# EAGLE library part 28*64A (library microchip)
CMOS EEPROM 64 K (8 K x 8), low voltage
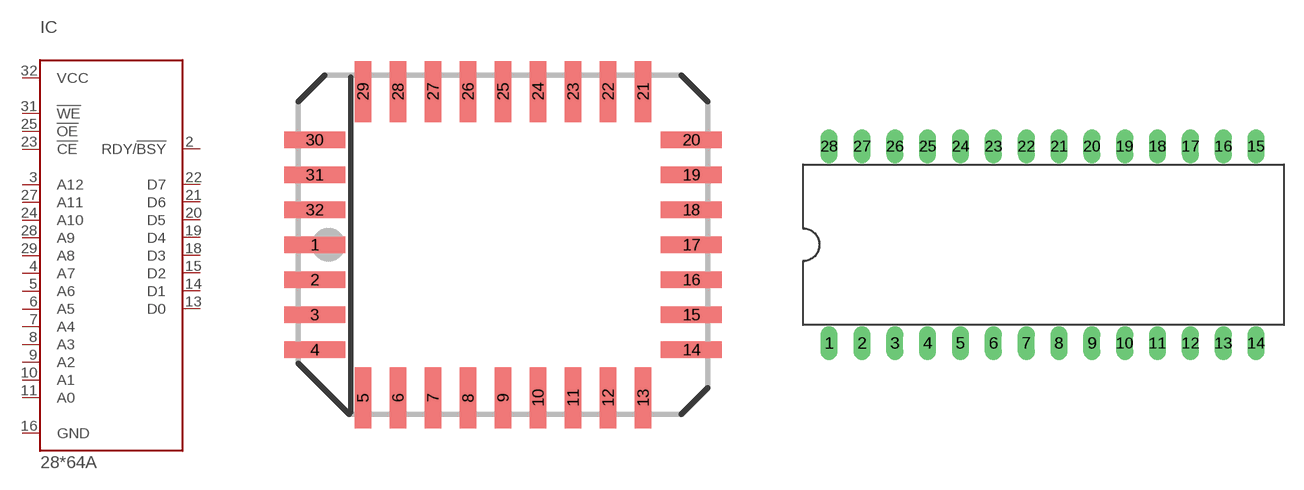
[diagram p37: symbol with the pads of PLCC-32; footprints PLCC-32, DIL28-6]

Designator prefix IC

## 28C64AL (MPN: CAT28C64BGI-12T; OC_FARNELL: 1718494; OC_NEWARK: 08R5439), 28VL64AL (OC_FARNELL: unknown; OC_NEWARK: unknown)  [PLCC-32]
2  RDY/!BSY  out
3  A12  in
4  A7  in
5  A6  in
6  A5  in
7  A4  in
8  A3  in
9  A2  in
10  A1  in
11  A0  in
13  D0  hiz
14  D1  hiz
15  D2  hiz
16  GND  pwr
18  D3  hiz
19  D4  hiz
20  D5  hiz
21  D6  hiz
22  D7  hiz
23  !CE  in
24  A10  in
25  !OE  in
27  A11  in
28  A9  in
29  A8  in
31  !WE  in
32  VCC  pwr

## 28C64AP (MPN: AT28C64B-15PU; OC_FARNELL: 1631144; OC_NEWARK: 96K6557), 28LV64AP (MPN: CAT28LV64LI-25; OC_FARNELL: unknown; OC_NEWARK: 06R0912)  [DIL28-6]
1  RDY/!BSY  out
2  A12  in
3  A7  in
4  A6  in
5  A5  in
6  A4  in
7  A3  in
8  A2  in
9  A1  in
10  A0  in
11  D0  hiz
12  D1  hiz
13  D2  hiz
14  GND  pwr
15  D3  hiz
16  D4  hiz
17  D5  hiz
18  D6  hiz
19  D7  hiz
20  !CE  in
21  A10  in
22  !OE  in
23  A11  in
24  A9  in
25  A8  in
27  !WE  in
28  VCC  pwr

## 28C64ASO (MPN: CAT28C64BWI-12; OC_FARNELL: 1718312; OC_NEWARK: 06R0739), 28LV64ASO (MPN: CAT28LV64W-25; OC_FARNELL: 1718338; OC_NEWARK: 06R0915)  [SO28W]
Pads as for DIL28-6

## 28C64AVS (OC_FARNELL: unknown; OC_NEWARK: unknown), 28LV64AVS (OC_FARNELL: unknown; OC_NEWARK: unknown)  [VSOP28-8X13]
Pads as for DIL28-6

## 28C64ATS (OC_FARNELL: unknown; OC_NEWARK: unknown), 28LV64ATS (MPN: CAT28LV64H13-20; OC_FARNELL: 1718417; OC_NEWARK: 06R0901)  [TSOP28]
1  !OE  in
2  A11  in
3  A9  in
4  A8  in
6  !WE  in
7  VCC  pwr
8  RDY/!BSY  out
9  A12  in
10  A7  in
11  A6  in
12  A5  in
13  A4  in
14  A3  in
15  A2  in
16  A1  in
17  A0  in
18  D0  hiz
19  D1  hiz
20  D2  hiz
21  GND  pwr
22  D3  hiz
23  D4  hiz
24  D5  hiz
25  D6  hiz
26  D7  hiz
27  !CE  in
28  A10  in

## Footprint PLCC-32 (pad centres in mm)
PLASTIC LEADED CHIP CARRIER rectangle, package type L
smd 2.2 x 0.6: 1 -6.83,0; 2 -6.83,-1.27; 3 -6.83,-2.54; 4 -6.83,-3.81; 14 6.83,-3.81; 15 6.83,-2.54; 16 6.83,-1.27; 17 6.83,0; 18 6.83,1.27; 19 6.83,2.54; 20 6.83,3.81; 30 -6.83,3.81; 31 -6.83,2.54; 32 -6.83,1.27
smd 0.6 x 2.2: 5 -5.08,-5.56; 6 -3.81,-5.56; 7 -2.54,-5.56; 8 -1.27,-5.56; 9 0,-5.56; 10 1.27,-5.56; 11 2.54,-5.56; 12 3.81,-5.56; 13 5.08,-5.56; 21 5.08,5.56; 22 3.81,5.56; 23 2.54,5.56; 24 1.27,5.56; 25 0,5.56; 26 -1.27,5.56; 27 -2.54,5.56; 28 -3.81,5.56; 29 -5.08,5.56

## Footprint DIL28-6 (pad centres in mm)
Dual In Line package type P
drill 0.813 long: 1 -16.51,-7.62; 2 -13.97,-7.62; 3 -11.43,-7.62; 4 -8.89,-7.62; 5 -6.35,-7.62; 6 -3.81,-7.62; 7 -1.27,-7.62; 8 1.27,-7.62; 9 3.81,-7.62; 10 6.35,-7.62; 11 8.89,-7.62; 12 11.43,-7.62; 13 13.97,-7.62; 14 16.51,-7.62; 15 16.51,7.62; 16 13.97,7.62; 17 11.43,7.62; 18 8.89,7.62; 19 6.35,7.62; 20 3.81,7.62; 21 1.27,7.62; 22 -1.27,7.62; 23 -3.81,7.62; 24 -6.35,7.62; 25 -8.89,7.62; 26 -11.43,7.62; 27 -13.97,7.62; 28 -16.51,7.62

## Footprint SO28W (pad centres in mm)
28-Lead Plastic Small Outline (SO) Wide, 300 mil Body (SOIC) Source: http://ww1.microchip.com/downloads/en/devicedoc/39632c.pdf
smd 0.65 x 1.7: 1 -7.62,-4.78; 2 -6.35,-4.78; 3 -5.08,-4.78; 4 -3.81,-4.78; 5 -2.54,-4.78; 6 -1.27,-4.78; 7 0,-4.78; 8 1.27,-4.78; 9 2.54,-4.78; 10 3.81,-4.78; 11 5.08,-4.78; 12 6.35,-4.78; 13 7.62,-4.78; 14 8.89,-4.78; 15 8.89,4.78; 16 7.62,4.78; 17 6.35,4.78; 18 5.08,4.78; 19 3.81,4.78; 20 2.54,4.78; 21 1.27,4.78; 22 0,4.78; 23 -1.27,4.78; 24 -2.54,4.78; 25 -3.81,4.78; 26 -5.08,4.78; 27 -6.35,4.78; 28 -7.62,4.78

## Footprint VSOP28-8X13 (pad centres in mm)
Very Small Outline Package 8 x 13.4 mm, package type VS
smd 0.3 x 1.1: 1 0.275,-6.45; 2 0.825,-6.45; 3 1.375,-6.45; 4 1.925,-6.45; 5 2.475,-6.45; 6 3.025,-6.45; 7 3.575,-6.45; 8 3.575,6.45; 9 3.025,6.45; 10 2.475,6.45; 11 1.925,6.45; 12 1.375,6.45; 13 0.825,6.45; 14 0.275,6.45; 15 -0.275,6.45; 16 -0.825,6.45; 17 -1.375,6.45; 18 -1.925,6.45; 19 -2.475,6.45; 20 -3.025,6.45; 21 -3.575,6.45; 22 -3.575,-6.45; 23 -3.025,-6.45; 24 -2.475,-6.45; 25 -1.925,-6.45; 26 -1.375,-6.45; 27 -0.825,-6.45; 28 -0.275,-6.45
